(* Logix 5000 AddOnInstructionDefinition export NORD_VFDcontrol_XU4_Inst110_111; software revision 24.02 *)

TYPE FI_Data_IN :
STRUCT
   ConnectionFaulted : BOOL;
   RunMode : BOOL;
   Data : INT[6];   // Actual Values
END_STRUCT
END_TYPE

TYPE FI_Data_OUT :
STRUCT
   Data : INT[6];   // Control Data
END_STRUCT
END_TYPE

ADD_ON_INSTRUCTION NORD_VFDcontrol_XU4_Inst110_111   (* revision 1.1, vendor NORD Drivesystems, ExecutePrescan *)
// Control Block for NORD VFD: CU4/TU4
// Revision note:
// Rev 1.1
// Better Ready Start Condition Logic
// Added Inhibited Output
// Added Fault Active Output
// Rev 1.0
// Connection to CU4/TU4-ETH (or EIP)
// Instances: Output 110/Input 111
// For VFD Series:
//    - BASE (SK 180E Series)
//    - FLEX (SK 200E Series)
//    - LINK (SK 250E-FDS Series)
// Allows for control of up to four (4) VFDs.
//    - FI_Control/Status may require Data Type change
// Access to remote IO on TU4 / CU4 modules via first word of process data.
VAR_IN_OUT
   FI_Status : _0342:CU4_ETH_15072931:I:0; {required}   // Input Data Map of VFD
   FI_Control : _0342:CU4_ETH_23BA2C07:O:0; {required}   // Output Data Map of VFD
END_VAR
VAR_OUTPUT
   TU_DI : SINT; {access Read Only, visible}   // Status of Digital Inputs on the EtherNet/IP Interface Module
END_VAR
VAR_INPUT
   TU_DO : SINT; {visible}   // Signals to the IO Ports on EtherNet/IP Interface Module
   Max_VFD_Number : SINT := 4;   // Maximum Number of VFDs on this specific node (1-4 for Instance 110/111)
   VFD_Number : SINT := 1; {visible}   // Number of VFD to control (1...Max_VFD_Number) for Instance 110/111)
   EnableFwd : BOOL; {visible}   // HIGH = Enable CW
   EnableRev : BOOL; {visible}   // HIGH = Enable CCW
   DisableVoltage : BOOL := 1; {visible}   // LOW = Output Voltage Disabled
   QuickStop : BOOL := 1; {visible}   // LOW = Emergency Stop Active
   FaultAckn : BOOL; {visible}   // Error / Fault Acknowledgement on Rising Edge
   ParameterSet : SINT := 1; {visible}   // Parameter Set 1-4, If less than 1 or higher than 4, Set 1 as active
   Activate32BitSetpoint : BOOL; {visible}   // HIGH = Activate 32Bit Setpoint combining Setpoint 2 and 3
   ControlWordBit8_P480_11 : BOOL; {visible}   // Control Word Bit 8 Function set in P480[11]
   ControlWordBit9_P480_12 : BOOL; {visible}   // Control Word Bit 9 Function set in P480[12]
   ControlWord : ALIAS FOR Control_Word; {access None, visible}   // Control Word Read Only Version
   Setpoint1 : INT; {visible}   // Setpoint 1 Function set in P546[1]
   Setpoint2 : INT; {visible}   // Setpoint 2 Function set in P546[2]
   Setpoint3 : INT; {visible}   // Setpoint 3 Function set in P546[3]
   Setpoint4 : INT;   // Setpoint 4 Reserved
   Setpoint5 : INT;   // Setpoint 5 Reserved
   Setpoint2_3_32 : DINT; {visible}   // 32 Bit Setpoint 2 & 3 combined for positioning
END_VAR
VAR_OUTPUT
   StatusWord : INT; {access Read Only, visible}   // Status Word
        .0   // Ready to Start
        .1   // Ready for Operation
        .2   // Operation Enabled
        .3   // Fault
        .4   // Voltage Enabled
        .5   // No Emergency Stop
        .6   // Starting Disabled
        .7   // Warning Active
        .8   // Setpoint Reached
        .9   // Bus Controller Active
        .10   // Function P481[9]
        .11   // Rotation Right Active
        .12   // Rotation Left Active
        .13   // Function P481[10]
        .14   // Parameter Set Bit 0
        .15   // Parameter Set Bit 1
   ActiveParameterSet : SINT; {access Read Only, visible}   // Displays active parameter set
   CommunicationOK : BOOL; {access Read Only, visible}   // HIGH = Communication is OK
   ReadyToStart : BOOL; {access Read Only, visible}   // HIGH = Drive Ready to Start
   VFD_Enabled : BOOL; {access Read Only, visible}   // HIGH = VFD is Enabled
   Inhibited : BOOL; {access Read Only, visible}   // VFD is Inhibited
   Warning : BOOL; {access Read Only, visible}   // HIGH = Drive has a warning
   Faulted : BOOL; {access Read Only, visible}   // HIGH = Drive Faulted
   FaultActive : BOOL; {access Read Only, visible}   // Fault Conditions are Currently Active
   StatusWordBit10_P481_9 : BOOL; {access Read Only, visible}   // Status Word Bit 10 Function set in P481[9]
   StatusWordBit13_P481_10 : BOOL; {access Read Only, visible}   // Status Word Bit 13 Function set in P481[10]
   ActualValue1 : INT; {access Read Only, visible}   // Actual Value 1 Function set in P543[1]
   ActualValue2 : INT; {access Read Only, visible}   // Actual Value 2 Function set in P543[2]
   ActualValue3 : INT; {access Read Only, visible}   // Actual Value 3 Function set in P543[3]
   ActualValue4 : INT; {access Read Only}   // Actual Value 4 Reserved
   ActualValue5 : INT; {access Read Only}   // Actual Value 5 Reserved
   ActualValue2_3_32 : DINT; {access Read Only, visible}   // 32 Bit Actual Value 2 & 3 Combined for Positioning
END_VAR
VAR
   Index : INT; {access None}   // Index of process data based on VFD address
   Control_Word : INT; {access None}   // Control Word
        .0   // Enable Operation
        .1   // Disable Voltage (Low level disables the output voltage of the drive and stops the VFD)
        .2   // Emergency Stop (Low level activates QuickStop mode and stops the VFD)
        .3   // Ready for Operation
        .4   // Enable Pulses
        .5   // Enable Ramp
        .6   // Enable Setpoint
        .7   // Error Acknowledge
        .8   // Function P480[11]
        .9   // Function P480[12]
        .10   // Control Data Valid
        .11   // Rotation Direction Clockwise
        .12   // Rotation Direction Counter-Clockwise
        .13   // Reserved
        .14   // Parameter Set Bit 0
        .15   // Parameter Set Bit 1
   Control : FI_Data_OUT; {access None}
   Status : FI_Data_IN; {access None}
   LowWordOf32BitSetpoint : DINT; {access None}
   Temporary_Variable_32BitSepoint : DINT; {access None}
   HighWordOf32BitSetpoint : DINT; {access None}
   FI_Control_Size : INT; {access None}   // Size of Output Process Data
   FI_Status_Size : INT; {access None}   // Size of Input Process Data
END_VAR

ROUTINE Logic   (* ladder *)
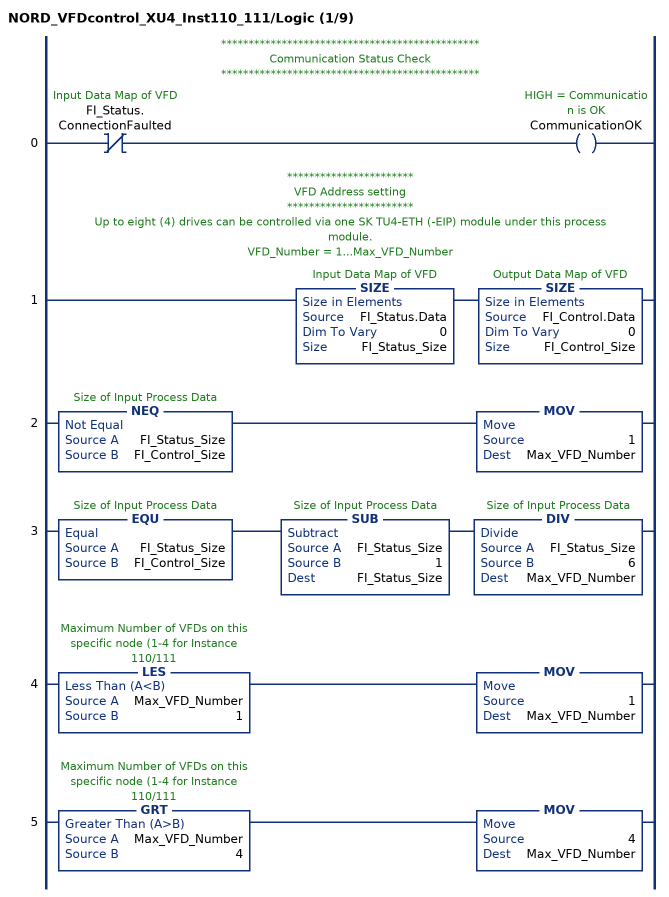
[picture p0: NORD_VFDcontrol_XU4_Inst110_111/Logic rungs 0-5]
   // ***********************************************
   // Communication Status Check
   // ***********************************************
   0: XIO(FI_Status.ConnectionFaulted)OTE(CommunicationOK);
   // ***********************
   // VFD Address setting
   // ***********************
   // Up to eight (4) drives can be controlled via one SK TU4-ETH (-EIP) module under this process module.
   // VFD_Number = 1...Max_VFD_Number
   1: SIZE(FI_Status.Data,0,FI_Status_Size)SIZE(FI_Control.Data,0,FI_Control_Size);
   2: NEQ(FI_Status_Size,FI_Control_Size)MOV(1,Max_VFD_Number);
   3: EQU(FI_Status_Size,FI_Control_Size)SUB(FI_Status_Size,1,FI_Status_Size)DIV(FI_Status_Size,6,Max_VFD_Number);
   4: LES(Max_VFD_Number,1)MOV(1,Max_VFD_Number);
   5: GRT(Max_VFD_Number,4)MOV(4,Max_VFD_Number);
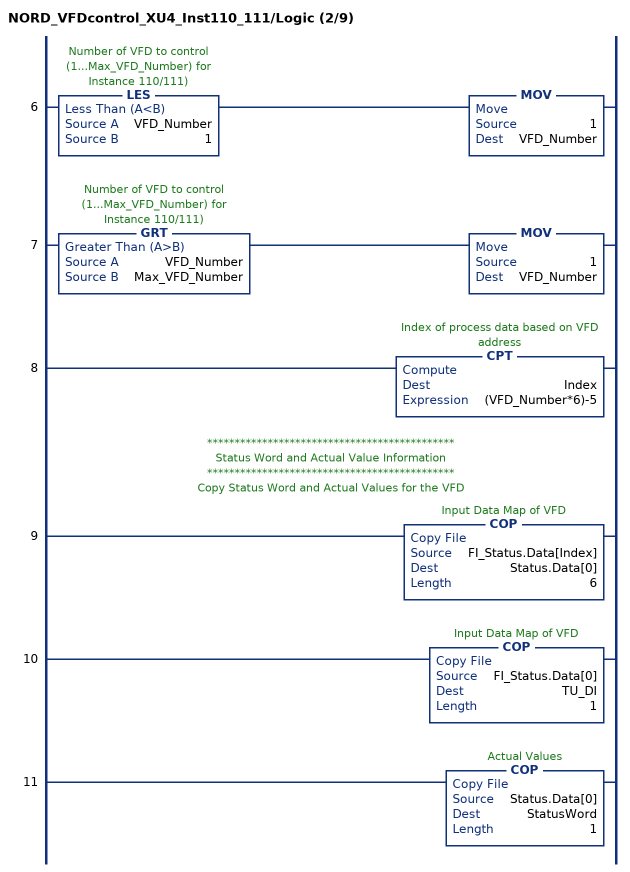
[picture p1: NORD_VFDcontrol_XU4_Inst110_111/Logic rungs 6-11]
   6: LES(VFD_Number,1)MOV(1,VFD_Number);
   7: GRT(VFD_Number,Max_VFD_Number)MOV(1,VFD_Number);
   8: CPT(Index,(VFD_Number*6)-5);
   // *********************************************
   // Status Word and Actual Value Information
   // *********************************************
   // Copy Status Word and Actual Values for the VFD
   9: COP(FI_Status.Data[Index],Status.Data[0],6);
   10: COP(FI_Status.Data[0],TU_DI,1);
   11: COP(Status.Data[0],StatusWord,1);
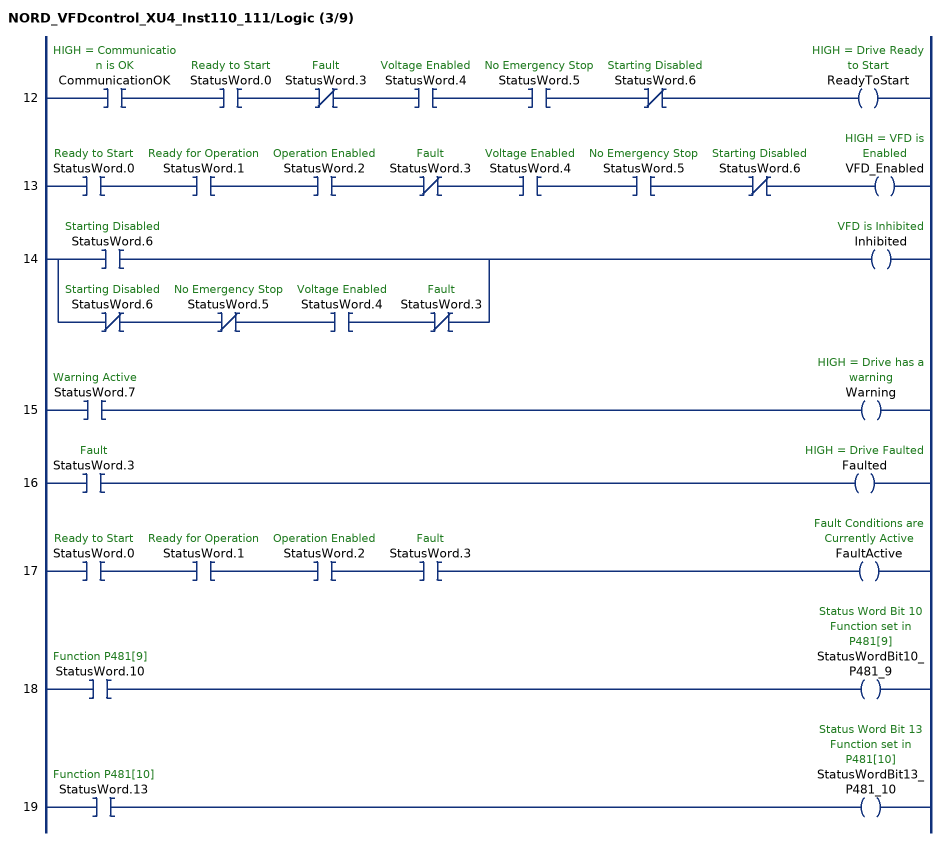
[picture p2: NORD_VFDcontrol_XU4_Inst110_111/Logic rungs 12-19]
   12: XIC(CommunicationOK)XIC(StatusWord.0)XIO(StatusWord.3)XIC(StatusWord.4)XIC(StatusWord.5)XIO(StatusWord.6)OTE(ReadyToStart);
   13: XIC(StatusWord.0)XIC(StatusWord.1)XIC(StatusWord.2)XIO(StatusWord.3)XIC(StatusWord.4)XIC(StatusWord.5)XIO(StatusWord.6)OTE(VFD_Enabled);
   14: [XIC(StatusWord.6) ,XIO(StatusWord.6) XIO(StatusWord.5) XIC(StatusWord.4) XIO(StatusWord.3) ]OTE(Inhibited);
   15: XIC(StatusWord.7)OTE(Warning);
   16: XIC(StatusWord.3)OTE(Faulted);
   17: XIC(StatusWord.0)XIC(StatusWord.1)XIC(StatusWord.2)XIC(StatusWord.3)OTE(FaultActive);
   18: XIC(StatusWord.10)OTE(StatusWordBit10_P481_9);
   19: XIC(StatusWord.13)OTE(StatusWordBit13_P481_10);
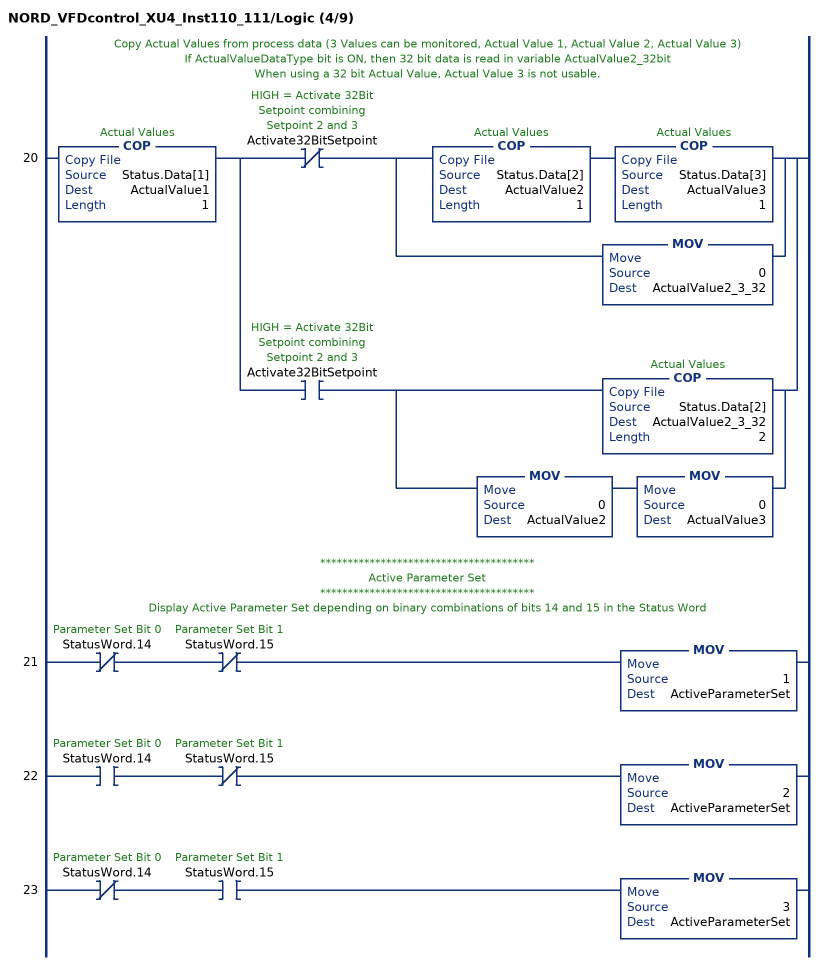
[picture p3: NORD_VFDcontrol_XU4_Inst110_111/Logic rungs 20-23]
   // Copy Actual Values from process data (3 Values can be monitored, Actual Value 1, Actual Value 2, Actual Value 3)
   // If ActualValueDataType bit is ON, then 32 bit data is read in variable ActualValue2_32bit
   // When using a 32 bit Actual Value, Actual Value 3 is not usable.
   20: COP(Status.Data[1],ActualValue1,1)[XIO(Activate32BitSetpoint) [COP(Status.Data[2],ActualValue2,1) COP(Status.Data[3],ActualValue3,1) ,MOV(0,ActualValue2_3_32) ] ,XIC(Activate32BitSetpoint) [COP(Status.Data[2],ActualValue2_3_32,2) ,MOV(0,ActualValue2) MOV(0,ActualValue3) ] ];
   // ***************************************
   // Active Parameter Set
   // ***************************************
   // Display Active Parameter Set depending on binary combinations of bits 14 and 15 in the Status Word
   21: XIO(StatusWord.14)XIO(StatusWord.15)MOV(1,ActiveParameterSet);
   22: XIC(StatusWord.14)XIO(StatusWord.15)MOV(2,ActiveParameterSet);
   23: XIO(StatusWord.14)XIC(StatusWord.15)MOV(3,ActiveParameterSet);
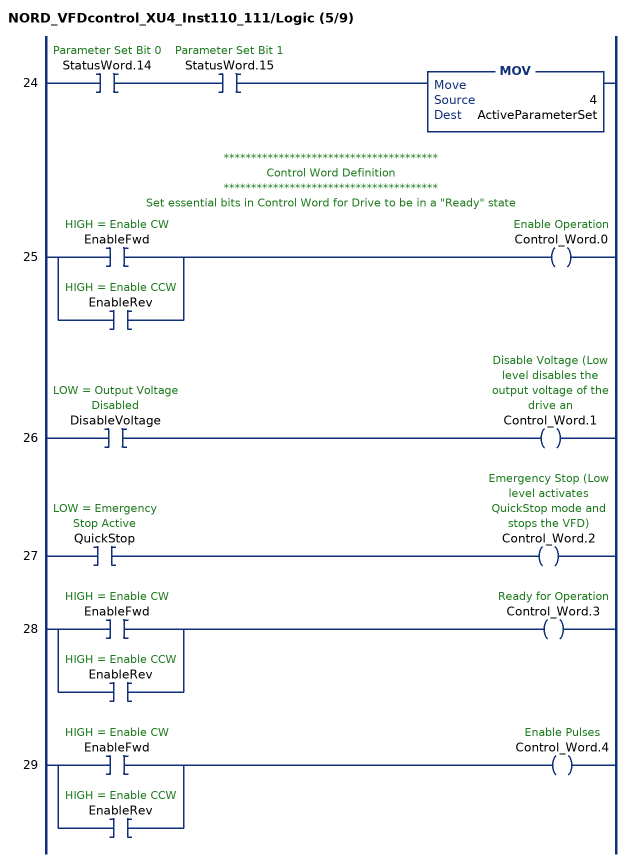
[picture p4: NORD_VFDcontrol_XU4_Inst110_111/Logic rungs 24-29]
   24: XIC(StatusWord.14)XIC(StatusWord.15)MOV(4,ActiveParameterSet);
   // ***************************************
   // Control Word Definition
   // ***************************************
   // Set essential bits in Control Word for Drive to be in a "Ready" state
   25: [XIC(EnableFwd) ,XIC(EnableRev) ]OTE(Control_Word.0);
   26: XIC(DisableVoltage)OTE(Control_Word.1);
   27: XIC(QuickStop)OTE(Control_Word.2);
   28: [XIC(EnableFwd) ,XIC(EnableRev) ]OTE(Control_Word.3);
   29: [XIC(EnableFwd) ,XIC(EnableRev) ]OTE(Control_Word.4);
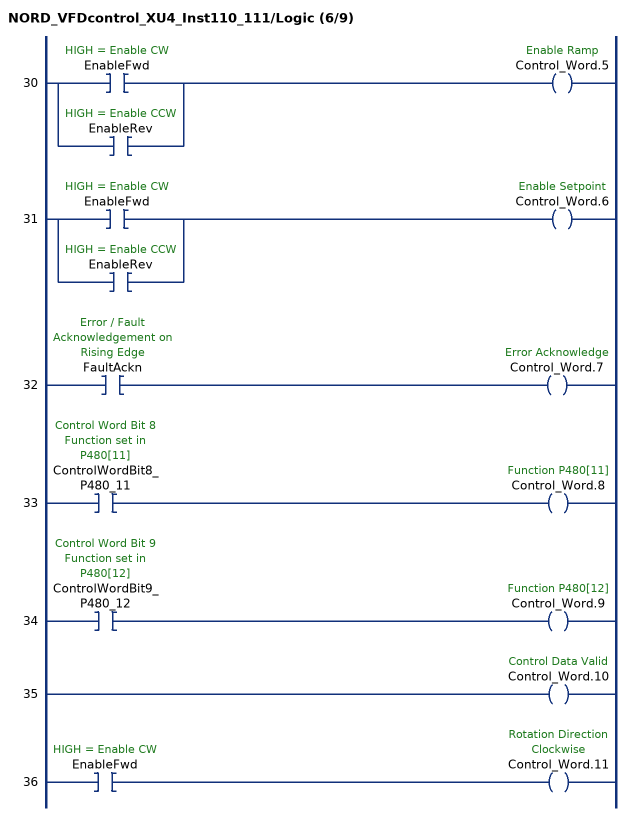
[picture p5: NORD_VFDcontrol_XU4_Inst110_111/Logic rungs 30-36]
   30: [XIC(EnableFwd) ,XIC(EnableRev) ]OTE(Control_Word.5);
   31: [XIC(EnableFwd) ,XIC(EnableRev) ]OTE(Control_Word.6);
   32: XIC(FaultAckn)OTE(Control_Word.7);
   33: XIC(ControlWordBit8_P480_11)OTE(Control_Word.8);
   34: XIC(ControlWordBit9_P480_12)OTE(Control_Word.9);
   35: OTE(Control_Word.10);
   36: XIC(EnableFwd)OTE(Control_Word.11);
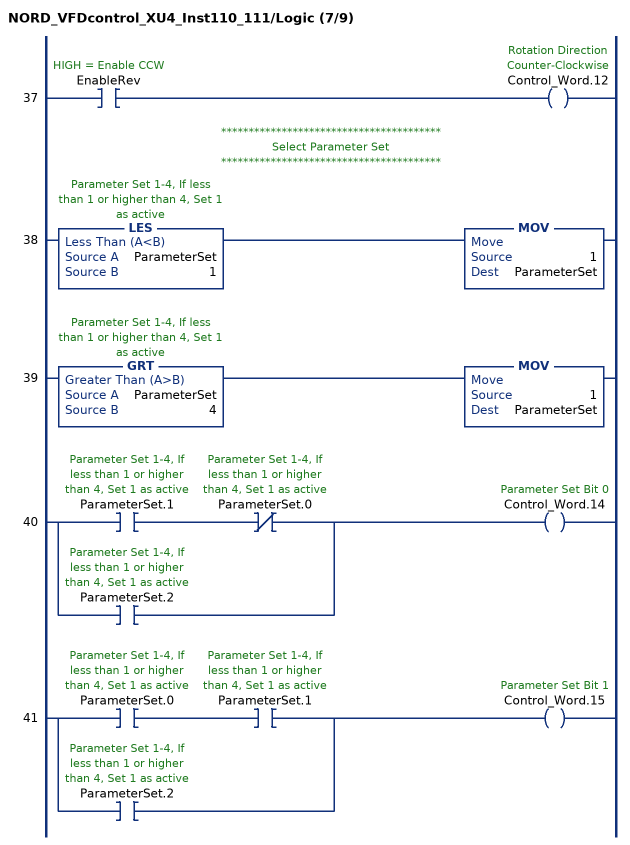
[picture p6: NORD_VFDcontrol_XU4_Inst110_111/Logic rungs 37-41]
   37: XIC(EnableRev)OTE(Control_Word.12);
   // ****************************************
   // Select Parameter Set
   // ****************************************
   38: LES(ParameterSet,1)MOV(1,ParameterSet);
   39: GRT(ParameterSet,4)MOV(1,ParameterSet);
   40: [XIC(ParameterSet.1) XIO(ParameterSet.0) ,XIC(ParameterSet.2) ]OTE(Control_Word.14);
   41: [XIC(ParameterSet.0) XIC(ParameterSet.1) ,XIC(ParameterSet.2) ]OTE(Control_Word.15);
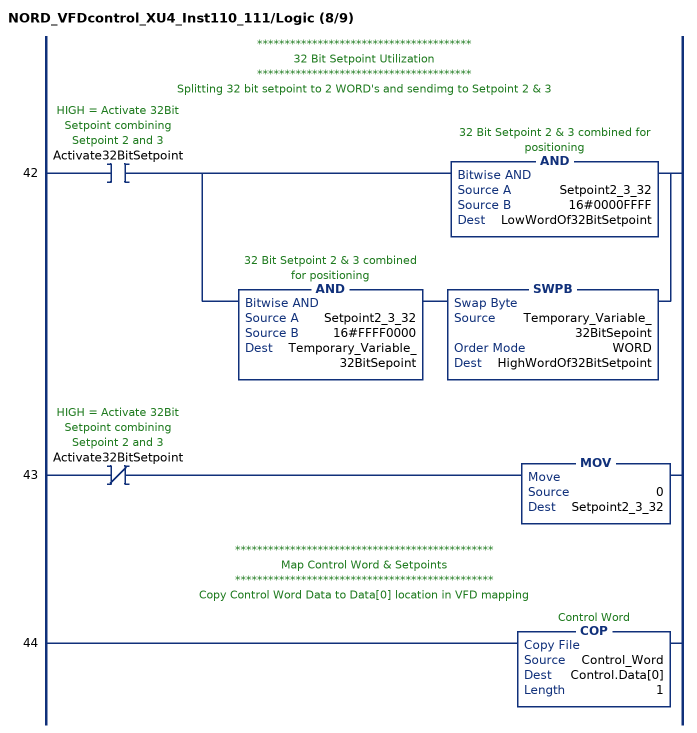
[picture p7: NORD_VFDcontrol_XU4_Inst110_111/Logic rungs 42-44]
   // ***************************************
   // 32 Bit Setpoint Utilization
   // ***************************************
   // Splitting 32 bit setpoint to 2 WORD's and sendimg to Setpoint 2 & 3
   42: XIC(Activate32BitSetpoint)[AND(Setpoint2_3_32,16#0000FFFF,LowWordOf32BitSetpoint) ,AND(Setpoint2_3_32,16#FFFF0000,Temporary_Variable_32BitSepoint) SWPB(Temporary_Variable_32BitSepoint,WORD,HighWordOf32BitSetpoint) ];
   43: XIO(Activate32BitSetpoint)MOV(0,Setpoint2_3_32);
   // ***********************************************
   // Map Control Word & Setpoints
   // ***********************************************
   // Copy Control Word Data to Data[0] location in VFD mapping
   44: COP(Control_Word,Control.Data[0],1);
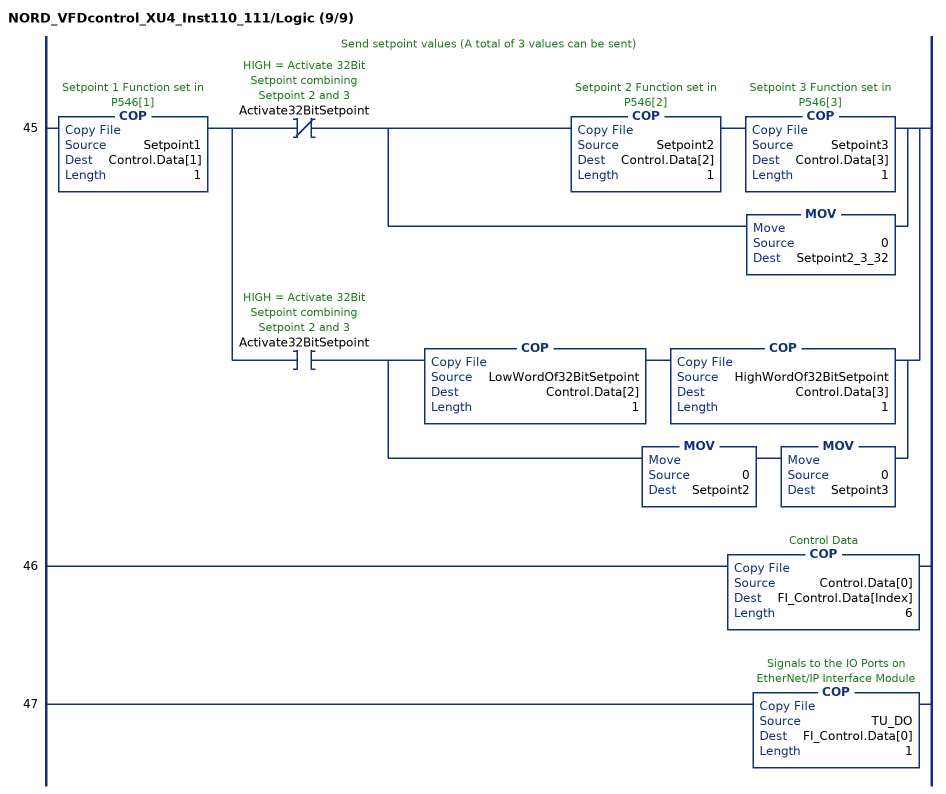
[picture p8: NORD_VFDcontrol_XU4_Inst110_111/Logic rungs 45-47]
   // Send setpoint values (A total of 3 values can be sent)
   45: COP(Setpoint1,Control.Data[1],1)[XIO(Activate32BitSetpoint) [COP(Setpoint2,Control.Data[2],1) COP(Setpoint3,Control.Data[3],1) ,MOV(0,Setpoint2_3_32) ] ,XIC(Activate32BitSetpoint) [COP(LowWordOf32BitSetpoint,Control.Data[2],1) COP(HighWordOf32BitSetpoint,Control.Data[3],1) ,MOV(0,Setpoint2) MOV(0,Setpoint3) ] ];
   46: COP(Control.Data[0],FI_Control.Data[Index],6);
   47: COP(TU_DO,FI_Control.Data[0],1);
END_ROUTINE

ROUTINE Prescan   (* ladder *)
// Executed prior to first scan of AOI
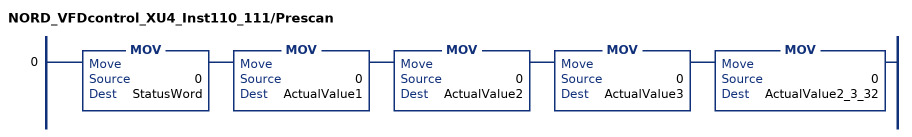
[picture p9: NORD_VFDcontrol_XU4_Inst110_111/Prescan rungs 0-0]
   0: MOV(0,StatusWord)MOV(0,ActualValue1)MOV(0,ActualValue2)MOV(0,ActualValue3)MOV(0,ActualValue2_3_32);
END_ROUTINE
END_ADD_ON_INSTRUCTION
